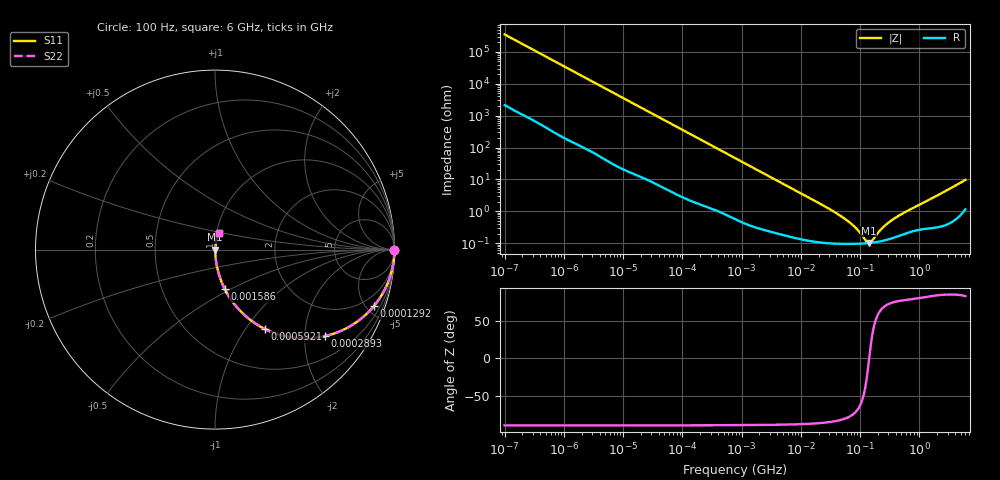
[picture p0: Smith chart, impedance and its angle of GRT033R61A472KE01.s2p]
!Murata Part Number: GRT033R61A472KE01
!These Parameters are Measured in Series Mode Connection
!Data Generated on Jun 19, 2026
!  o--ll--o
!Port1  Port2
!  o------o
!Operation Temp=25[degC], DC Bias Voltage=0[V]
!Freq. Start=100[Hz] Stop=6[GHz] 401[Steps]
# Hz S RI R 50
!Freq.(Hz) S11(Real) S11(Imag) S21(Real) S21(Imag) S12(Real) S12(Imag) S22(Real) S22(Imag)
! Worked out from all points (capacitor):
!   401 points, 100 Hz to 6 GHz, reference 50 ohm
!   read as one part in series: C = 4.52 nF near 109 Hz
!   lowest |Z| = 102 mohm at 139.6 MHz (marker M1)
!   series resonance near 142.6 MHz, so ESL is about 280 pH
!   S11 on the Smith chart (normalised r, x): 100 Hz: open; 129.2 kHz: 1.04, -5.59; 289.3 kHz: 1.03, -2.51; 592.1 kHz: 1.01, -1.23; 1.586 MHz: 1.01, -0.46; 6 GHz: 1.02, +0.19
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100  1 -0.000284  1.8e-06 0.000284  1.8e-06 0.000284  1 -0.000284
2008  0.9999 -0.00565  6.59e-05 0.00565  6.59e-05 0.00565  0.9999 -0.00565
12592  0.9986 -0.0351  0.00145 0.0351  0.00145 0.0351  0.9986 -0.0351
40335  0.9868 -0.1106  0.0132 0.1106  0.0132 0.1106  0.9868 -0.1106
129199  0.8847 -0.3154  0.1153 0.3154  0.1153 0.3154  0.8847 -0.3154
193316  0.7761 -0.4124  0.2239 0.4124  0.2239 0.4124  0.7761 -0.4124
289253  0.6104 -0.4826  0.3896 0.4826  0.3896 0.4826  0.6104 -0.4826
413847  0.4367 -0.4904  0.5633 0.4904  0.5633 0.4904  0.4367 -0.4904
592111  0.2775 -0.4419  0.7225 0.4419  0.7225 0.4419  0.2775 -0.4419
774597  0.1851 -0.3824  0.8149 0.3824  0.8149 0.3824  0.1851 -0.3824
1585629  0.0536 -0.2183  0.9464 0.2183  0.9464 0.2183  0.0536 -0.2183
4246196  0.00942 -0.086  0.9906 0.086  0.9906 0.086  0.00942 -0.086
1.555665e7  0.0017 -0.0237  0.9983 0.0237  0.9983 0.0237  0.0017 -0.0237
6.233367e7  0.000972 -0.00486  0.999 0.00486  0.999 0.00486  0.000972 -0.00486
8.527865e7  0.000965 -0.00282  0.999 0.00282  0.999 0.00282  0.000965 -0.00282
1.275994e8  0.000997 -0.00058  0.999 0.00058  0.999 0.00058  0.000997 -0.00058
1.395531e8  0.00101 -0.00011  0.999 0.00011  0.999 0.00011  0.00101 -0.00011
1.596157e8  0.00104 0.000592  0.999 -0.000592  0.999 -0.000592  0.00104 0.000592
2.283698e8  0.00117 0.00253  0.9988 -0.00253  0.9988 -0.00253  0.00117 0.00253
3.124326e8  0.00137 0.00443  0.9986 -0.00443  0.9986 -0.00443  0.00137 0.00443
5.59173e8  0.00202 0.00891  0.998 -0.00891  0.998 -0.00891  0.00202 0.00891
6e9  0.0203 0.093  0.9797 -0.093  0.9797 -0.093  0.0203 0.093
